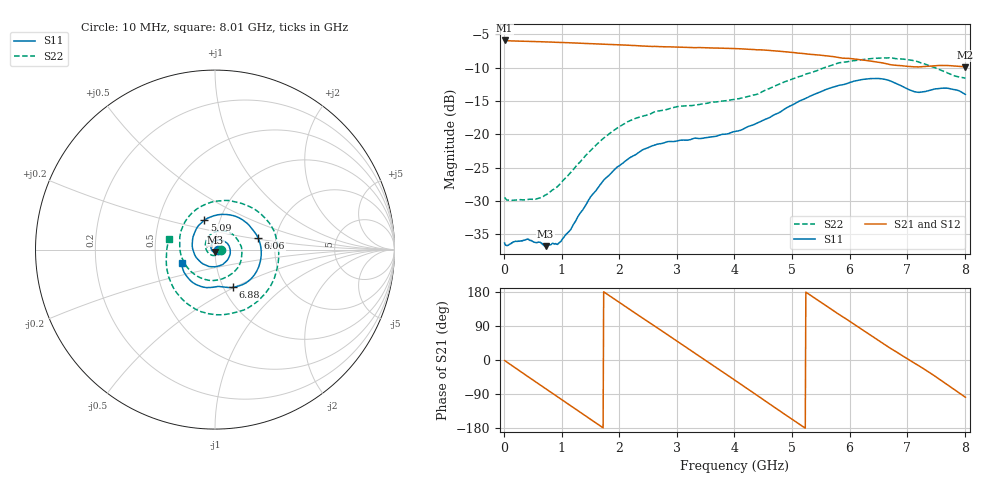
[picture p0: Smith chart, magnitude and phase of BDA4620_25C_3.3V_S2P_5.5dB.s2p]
!Agilent Technologies,E5071B,MY42404982,A.09.10
!Date: Wed May 06 08:49:28 2026
!Data & Calibration Information:
!Freq	S11:SOLT2(ON)	S21:SOLT2(ON)	S12:SOLT2(ON)	S22:SOLT2(ON)
# Hz S RI R 50
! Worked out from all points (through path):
!   801 points, 10 MHz to 8.01 GHz, reference 50 ohm
!   highest |S21| = -5.95 dB at 10 MHz (marker M1); lowest = -9.9 dB at 8.01 GHz (marker M2)
!   group delay of S21, straight-line fit = 284 ps
!   lowest |S11| = -36.8 dB at 720 MHz (marker M3), VSWR 1.03, Z = 50.2 - j1.44 ohm
!   |S11| at or under -10 dB: start of sweep to end of sweep
!   |S22| runs from -29.9 to -8.5 dB; largest |S21 - S12| = 0.002
!   S11 on the Smith chart (normalised r, x): 10 MHz: 1.03, -0.00; 5.09 GHz: 0.84, +0.28; 6.06 GHz: 1.61, +0.23; 6.88 GHz: 1.10, -0.49; 8.01 GHz: 0.68, -0.10
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1e7  0.0153 -0.000906  0.5041 -0.0109  0.5047 -0.0111  0.0336 -0.00263
3.4e8  0.0142 -0.00756  0.403 -0.2917  0.403 -0.2922  0.0213 -0.0242
7.2e8  0.00217 -0.0143  0.1222 -0.4764  0.1222 -0.477  -0.0134 -0.0324
9.7e8  -0.0113 -0.0106  -0.098 -0.4773  -0.0982 -0.4783  -0.039 -0.0164
1.35e9  -0.0228 0.0137  -0.3733 -0.3024  -0.3734 -0.3026  -0.0522 0.0372
1.64e9  -0.0128 0.0381  -0.4684 -0.0758  -0.4688 -0.0756  -0.0268 0.082
1.93e9  0.0137 0.0533  -0.4383 0.1651  -0.439 0.1652  0.0276 0.1052
2.32e9  0.058 0.0427  -0.2255 0.4016  -0.2261 0.4017  0.1101 0.0749
2.68e9  0.0846 0.00163  0.0563 0.4501  0.0566 0.4507  0.1493 -0.00249
2.99e9  0.0771 -0.0443  0.2813 0.3522  0.2819 0.3521  0.137 -0.0835
3.38e9  0.0349 -0.0859  0.4369 0.0896  0.4372 0.0886  0.0508 -0.1589
3.69e9  -0.0161 -0.0954  0.4145 -0.1538  0.4143 -0.1547  -0.0516 -0.1668
4.01e9  -0.0722 -0.076  0.2605 -0.3521  0.26 -0.3528  -0.1497 -0.1051
4.51e9  -0.1266 0.0185  -0.1138 -0.4124  -0.1145 -0.4124  -0.1943 0.0832
5.09e9  -0.0597 0.1632  -0.3935 -0.1014  -0.3939 -0.1008  -0.00696 0.2675
5.35e9  0.0213 0.1951  -0.3872 0.0828  -0.3871 0.0834  0.1227 0.2639
5.72e9  0.1535 0.166  -0.245 0.2922  -0.2447 0.293  0.2877 0.1658
6.06e9  0.2399 0.0658  -0.0373 0.3654  -0.0368 0.366  0.3551 -0.016
6.68e9  0.1727 -0.1855  0.2787 0.1841  0.2799 0.1841  0.1901 -0.3215
6.88e9  0.0985 -0.2102  0.3158 0.0834  0.3171 0.0832  0.0764 -0.3585
7.46e9  -0.0497 -0.2115  0.2476 -0.2109  0.2476 -0.2121  -0.2242 -0.2252
8.01e9  -0.1847 -0.0735  -0.0454 -0.3151  -0.046 -0.316  -0.2562 0.0587
